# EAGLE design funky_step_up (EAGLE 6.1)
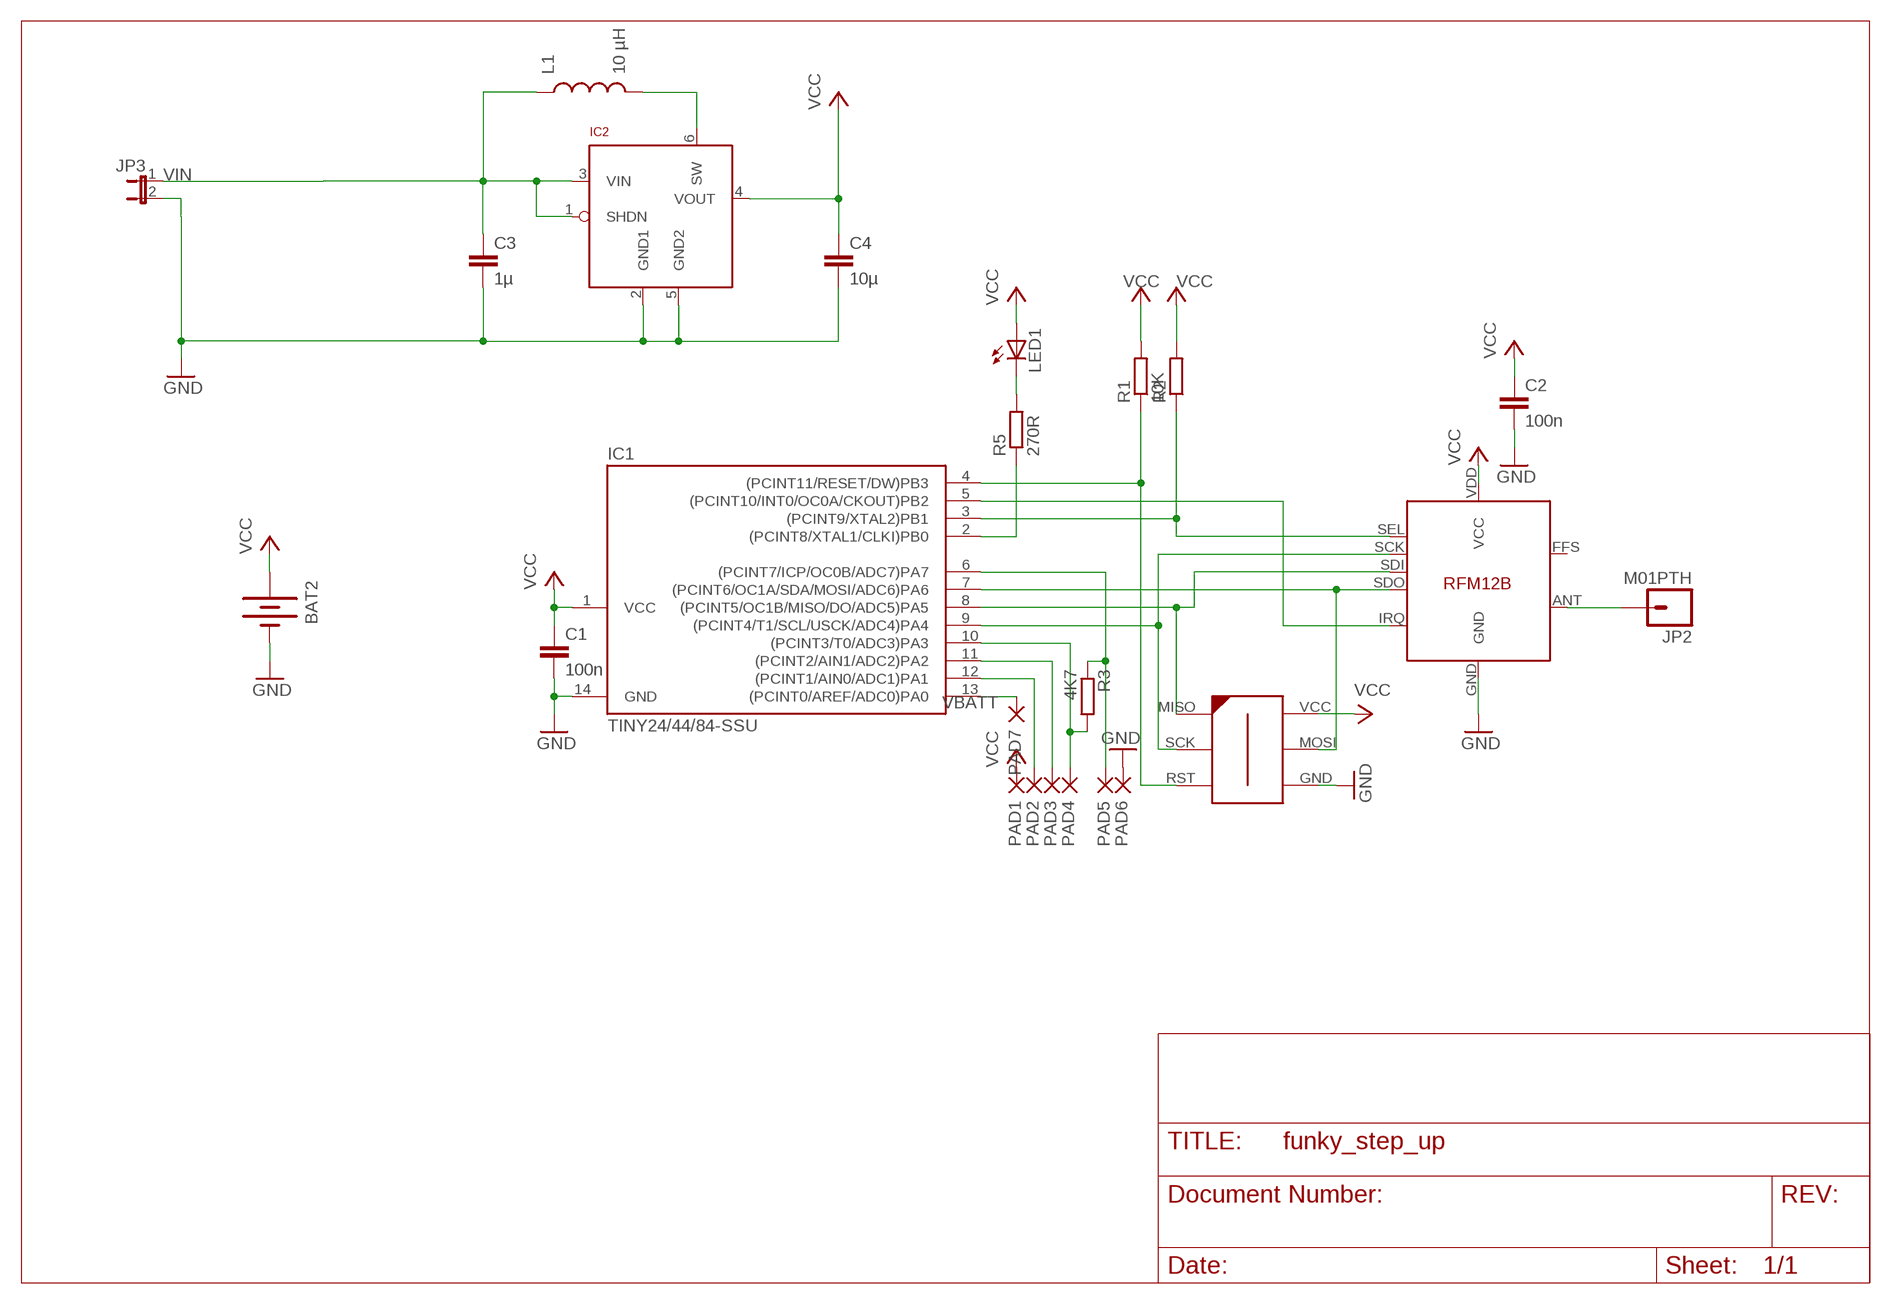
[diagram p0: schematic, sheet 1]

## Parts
BAT2  BATTERY20PTH  [BATTCOM_20MM_PTH]
C1  100n  C-EUC0603K  [C0603K]
C2  100n  C-EUC0603K  [C0603K]
C3  1µ  CAP0603-CAP  [0603-CAP]
C4  10µ  CAP0805  [0805]
IC1  TINY24/44/84-SSU  [SOIC14]
IC2  LTC3525  [SC70]
JP2  M01PTH  [1X01]
JP3  JUMPER-2PTH  [1X02]
L1  10 µH  INDUCTOR1210  [1210]
LED1  LED0603  [LED-0603]
PAD1  SMD2  [SMD1,27-2,54]
PAD2  SMD2  [SMD1,27-2,54]
PAD3  SMD2  [SMD1,27-2,54]
PAD4  SMD2  [SMD1,27-2,54]
PAD5  SMD2  [SMD1,27-2,54]
PAD6  SMD2  [SMD1,27-2,54]
PAD7  SMD2  [SMD1,27-2,54]
R1  10K  R-EU_R0603  [R0603]
R2  R-EU_R0603  [R0603]
R3  4K7  R-EU_R0603  [R0603]
R5  270R  R-EU_R0603  [R0603]
U$1  RFM12B  [RFM12B]
U$2  AVR-ISP-6-EDGE  [6PAD_ISP]

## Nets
GND: BAT2.2(-) C1.2 C2.2 C3.2 C4.2 IC1.14(GND) IC2.2(GND1) IC2.5(GND2) JP3.2 PAD6.1(P) U$1.GND U$2.GND
N$1: IC1.4((PCINT11/RESET/DW)PB3) R1.1 U$2.RST
N$2: IC1.3((PCINT9/XTAL2)PB1) R2.1 U$1.SEL
N$3: JP2.1 U$1.ANT
N$4: IC1.9((PCINT4/T1/SCL/USCK/ADC4)PA4) U$1.SCK U$2.SCK
N$5: IC1.8((PCINT5/OC1B/MISO/DO/ADC5)PA5) U$1.SDI U$2.MISO
N$6: IC1.7((PCINT6/OC1A/SDA/MOSI/ADC6)PA6) U$1.SDO U$2.MOSI
N$7: IC1.5((PCINT10/INT0/OC0A/CKOUT)PB2) U$1.IRQ
N$8: IC1.6((PCINT7/ICP/OC0B/ADC7)PA7) PAD5.1(P) R3.1
N$9: IC1.10((PCINT3/T0/ADC3)PA3) PAD4.1(P) R3.2
N$10: IC1.11((PCINT2/AIN1/ADC2)PA2) PAD3.1(P)
N$11: IC1.12((PCINT1/AIN0/ADC1)PA1) PAD2.1(P)
N$12: LED1.C R5.2
N$13 [power]: IC2.6(SW) L1.2
N$14: IC1.2((PCINT8/XTAL1/CLKI)PB0) R5.1
VBATT: IC1.13((PCINT0/AREF/ADC0)PA0) PAD7.1(P)
VCC: BAT2.1(+) C1.1 C2.1 C4.1 IC1.1(VCC) IC2.4(VOUT) LED1.A PAD1.1(P) R1.2 R2.2 U$1.VDD(VCC) U$2.VCC
VIN: C3.1 IC2.1(SHDN) IC2.3(VIN) JP3.1 L1.1
Unconnected: U$1.FFS

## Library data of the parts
BAT2 = SparkFun:BATTERY: Battery Holders
C1 C2 = rcl:C-EU: CAPACITOR, European symbol
C3 C4 = SparkFun:CAP: Capacitor
IC1 = avr-7:TINY24/44/84
IC2 = JeeLabs:LTC3525
JP2 = SparkFun:M01: Header 1
JP3 = SparkFun:JUMPER-2: Jumper
L1 = SparkFun:INDUCTOR: Inductors
LED1 = SparkFun:LED: LEDs
PAD1-PAD7 = wirepad:SMD2: SMD PAD
R1-R3 R5 = resistor:R-EU_: RESISTOR, European symbol
U$1 = JeeParts:RFM12B
U$2 = avr-7:AVR-ISP-6-EDGE: 6 pin edge connector for ISP with ATMEL MCUs. Developed by Craig Moates (craig at moates dot net). Library by David Blundell (blundar at gmail dot com). Often, even a 6 pin header is really inconvenient for board layout and/or production. This SMD-only header is our de-facto standard for using an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

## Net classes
1 power: width 0.305 mm, clearance 0.203 mm

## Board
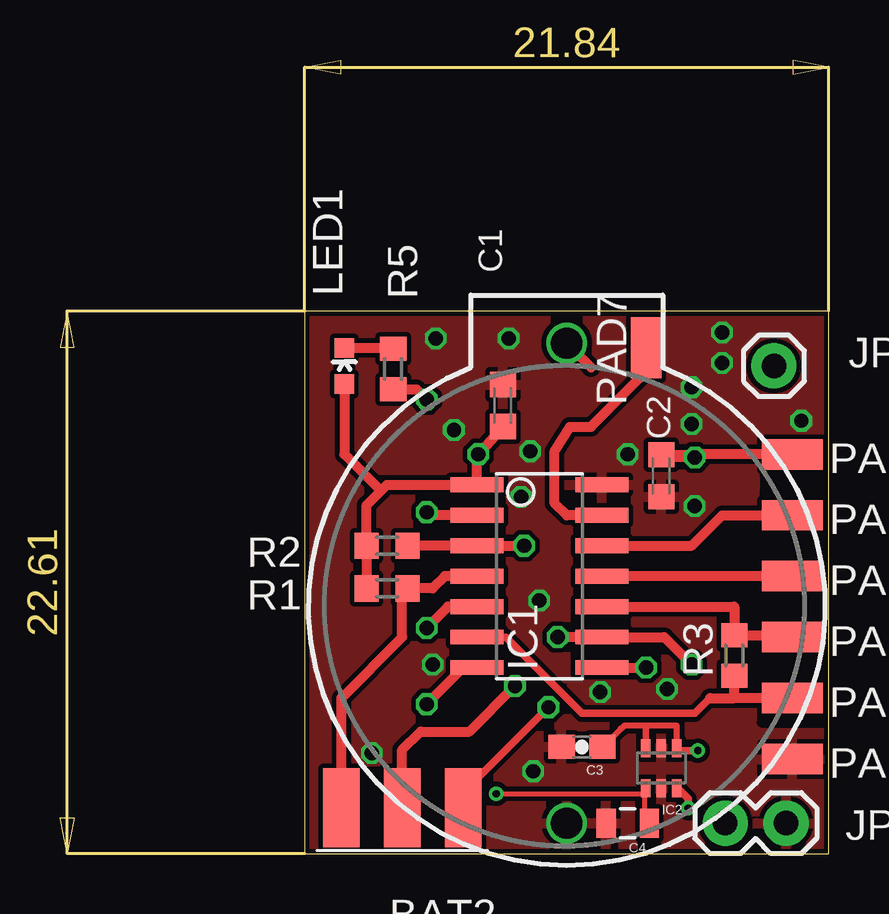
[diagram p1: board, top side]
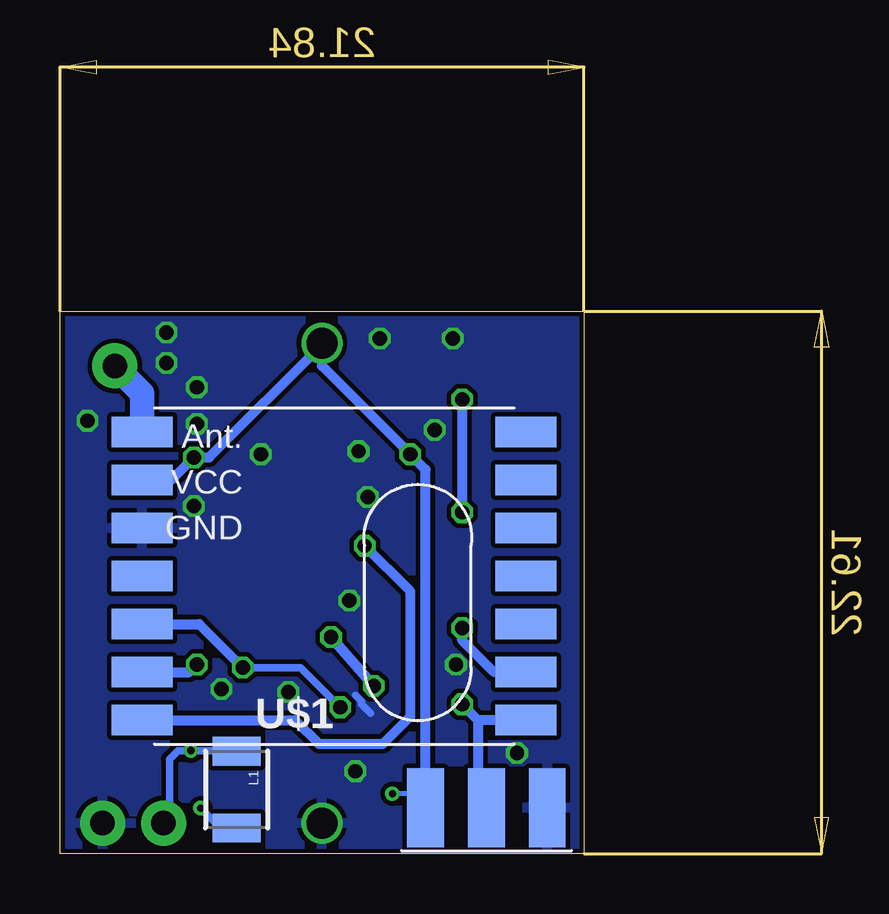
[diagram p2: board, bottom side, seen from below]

Size 32.05 x 33.07 mm. Coordinates in mm from the lower left corner, seen from the top.
Outline: 10.21,0 32.05,0 32.05,22.61 10.21,22.61 10.21,0
Copper layers (1*16): Top 0.035mm / dielectric 1.5mm / Bottom 0.035mm
Design rules: minimum track width 0.2mm, minimum drill 0.3mm, track to track 0.2mm, track to pad 0.2mm, pad to pad 0.2mm, via to via 0.2mm, smd to smd 0.2mm, copper to edge 0.2mm, drill to drill 0.2mm, minimum pad ring 0.2mm, minimum via ring 0.15mm, stop-mask expansion 0.075mm, vias tented up to drill 0mil, thermal gap 0.2mm
tRestrict: 5 lines
bRestrict: 2 lines

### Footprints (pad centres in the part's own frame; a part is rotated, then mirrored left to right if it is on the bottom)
BATTCOM_20MM_PTH = drill 1.3: 1 20,0; 2 0,0
C0603K = smd 1.05 x 1.08: 1 -0.875,0; 2 0.875,0
0603-CAP = smd 1.1 x 1: 1 -0.85,0; 2 0.85,0
0805 = smd 0.8 x 1.2: 1 -0.9,0; 2 0.9,0
SOIC14 = smd 0.61 x 2.21: 1 -3.81,-2.603; 2 -2.54,-2.603; 3 -1.27,-2.603; 4 0,-2.603; 5 1.27,-2.603; 6 2.54,-2.603; 7 3.81,-2.603; 8 3.81,2.603; 9 2.54,2.603; 10 1.27,2.603; 11 0,2.603; 12 -1.27,2.603; 13 -2.54,2.603; 14 -3.81,2.603
SC70 = smd 0.4 x 0.75: 1 -0.65,-0.825; 2 0,-0.825; 3 0.65,-0.825; 4 0.65,0.825; 5 0,0.825; 6 -0.65,0.825
1X01 = drill 1.016 pad 1.88: 1 0,0
1X02 = drill 1.016 pad 1.88: 1 0,0; 2 2.54,0
1210 = smd 1.2 x 2: 1 -1.6,0; 2 1.6,0
LED-0603 = smd 0.8 x 0.8: A 0,-0.75; C 0,0.75
SMD1,27-2,54 = smd 1.27 x 2.54: 1 0,0
R0603 = smd 1 x 1.1: 1 -0.85,0; 2 0.85,0
RFM12B = smd 2.54 x 1.27: ANT 8,-6; FFS -8,2; GND 8,-2; IRQ -8,4; P$8 -8,0; P$9 -8,-2; P$10 -8,-4; P$12 -8,-6; P$16 8,0; SCK 8,4; SDI 8,2; SDO -8,6; SEL 8,6; VDD 8,-4
6PAD_ISP = smd 1.524 x 3.302 bottom: GND 2.54,0; MOSI 0,0; VCC -2.54,0 | smd 1.524 x 3.302: MISO -2.54,0; RST 2.54,0; SCK 0,0

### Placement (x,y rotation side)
BAT2  21.13,1.27 90 top
C1  18.46,18.67 90 top
C2  25.07,15.75 270 top
C3  21.76,4.45 180 top
C4  23.67,1.27 180 top
IC1  19.98,11.56 270 top
IC2  25.07,3.56 180 top
JP2  29.76,20.32 0 top
JP3  27.73,1.27 0 top
L1  24.68,2.67 270 bottom
LED1  11.86,20.32 0 top
PAD1  30.53,16.64 90 top
PAD2  30.53,14.1 90 top
PAD3  30.53,11.56 90 top
PAD4  30.53,9.02 90 top
PAD5  30.53,6.48 90 top
PAD6  30.53,3.94 90 top
PAD7  24.43,21.08 0 top
R1  13.64,11.05 180 top
R2  13.64,12.83 180 top
R3  28.11,8.25 90 top
R5  13.89,20.19 90 top
U$1  20.62,11.56 180 bottom
U$2  14.27,1.9 180 top

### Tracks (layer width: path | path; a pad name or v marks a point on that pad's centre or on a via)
GND  (via drill 0.6)
  Bottom 0.305: 19.73,6.6 19.48,6.35 19.48,6.22 19.1,5.84
  other vias: 27.61,21.72 16.43,17.65 18.72,21.46 19.6,16.76 19.98,10.54 19.22,14.86 26.46,14.48 25.32,6.86 30.91,18.03 23.67,16.64 26.34,17.91 26.34,19.43 27.61,20.45 22.53,6.73 15.67,21.46 13,4.19 15.54,7.87 19.73,3.43
  pour Top: 10.46,22.48 31.8,22.48 31.8,0.13 10.46,0.13
  pour Bottom: 10.46,22.48 31.8,22.48 31.8,0.13 10.46,0.13
N$1
  Top 0.406: U$2.RST 11.73,6.48 14.27,9.02 14.27,11.34 R1.1 15.54,11.05 16.05,11.56 IC1.4
N$2  (via drill 0.6)
  Top 0.406: v19.35,12.83 IC1.3 R2.1
  Bottom 0.406: U$1.SEL 22.24,5.56 21.26,4.57 18.59,4.57 17.45,5.71 17.45,10.92 v19.35,12.83
N$3
  Bottom 1.016: U$1.ANT 28.62,19.18 JP2.1
N$4  (via drill 0.6)
  Top 0.406: v20.75,9.02 IC1.9 25.19,9.02 v26.34,7.87 | U$2.SCK 14.27,4.32 15.03,5.08 17.06,5.08 v18.97,6.99
  Bottom 0.406: v20.75,9.02 v18.97,6.99 | U$1.SCK 26.65,7.56 v26.34,7.87
N$5  (via drill 0.6)
  Top 0.305: U$2.MISO 16.81,2.54 v20.37,6.1
  Top 0.406: IC1.8 v24.43,7.75
  Bottom 0.305: v24.43,7.75 22.02,7.75 v20.37,6.1
  Bottom 0.406: U$1.SDI 26.24,9.56 v24.43,7.75
N$6  (via drill 0.6)
  Top 0.406: IC1.7 16.81,7.75 v15.29,6.22
  Bottom 0.406: U$1.SDO 14.62,5.56 | 14.62,5.56 v15.29,6.22 | 14.62,5.56 14.62,1.75 U$2.MOSI
N$7  (via drill 0.6)
  Top 0.406: IC1.5 16.18,10.29 v15.29,9.4
  Bottom 0.406: U$1.IRQ 13.95,7.56 15.29,8.89 v15.29,9.4
N$8
  Top 0.305: IC1.6 18.59,9.02 21.76,5.84 25.7,5.84 26.46,5.84 27.1,6.48
  Top 0.406: PAD5.1 28.11,6.48 | 28.11,6.48 R3.1 28.11,6.48 | 27.1,6.48 28.11,6.48
N$9
  Top 0.406: IC1.10 28.11,10.29 R3.2 30.53,9.11 PAD4.1
N$10
  Top 0.406: PAD3.1 IC1.11
N$11
  Top 0.406: IC1.12 26.34,12.83 27.61,14.1 PAD2.1
N$12
  Top 0.406: LED1.C 13.86,21.07 R5.2
N$13  (via drill 0.3)
  Top 0.305: v26.19,1.89 26.19,2.29 25.79,2.69 IC2.6
  Bottom 0.305: v26.19,1.89 25.39,1.09 24.79,1.09 L1.2
N$14  (via drill 0.6)
  Top 0.406: IC1.2 15.29,14.1 v15.29,14.22 | R5.1 14.87,19.34 v15.29,18.92
  Bottom 0.406: v15.29,18.92 v15.29,14.22 15.29,14.1
VBATT
  Top 0.406: IC1.13 21.13,14.1 20.62,14.61 20.62,16.76 21.26,17.78 22.14,17.78 24.43,20.07 PAD7.1 24.3,20.96 24.3,20.83
VCC  (via drill 0.3, 0.6)
  Top 0.2: 24.39,2.49 24.39,1.29 C4.1 | 24.39,2.49 24.39,2.69 IC2.4 24.39,2.49 | v18.19,2.49 24.39,2.49
  Top 0.406: 13.38,15.11 12.79,14.52 R2.2 R1.2 | 13.38,15.11 13.64,15.37 IC1.1 17.38,16.57 v17.45,16.64 C1.1 | 22.14,20.25 BAT2.1 | v26.46,16.51 25.18,16.51 C2.1 26.35,16.62 v26.46,16.51 | LED1.A 11.86,16.64 13.38,15.11 | PAD1.1 26.59,16.64 v26.46,16.51
  Bottom 0.2: v18.19,2.49 16.99,2.49 U$2.VCC
  Bottom 0.406: U$2.VCC 16.81,16 v17.45,16.64 21.13,20.32 21.13,21.21 | BAT2.1 21.13,21.21 | U$1.VDD 27.42,15.56 v26.46,16.51 25.83,16.51 21.13,21.21
VIN  (via drill 0.3)
  Top 0.254: IC2.1 25.71,5.32 25.7,5.33 24.43,5.33 | 24.43,5.33 24.43,4.49 | 24.43,4.49 24.43,4.45 24.43,4.49 | 24.43,4.49 24.43,5.33 | 24.43,5.33 23.54,5.33 23.41,5.21 23.38,5.21 C3.1
  Top 0.305: IC2.3 24.39,4.49 24.43,4.49 | v26.59,4.29 25.79,4.29 IC2.1
  Bottom 0.305: L1.1 24.79,4.29 v26.59,4.29 27.12,4.29 27.48,3.94 27.48,1.52 JP3.1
